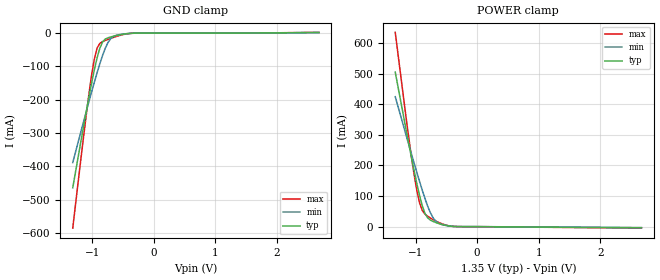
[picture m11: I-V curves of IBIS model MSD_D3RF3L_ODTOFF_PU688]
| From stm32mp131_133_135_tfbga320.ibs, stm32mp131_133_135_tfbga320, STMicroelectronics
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[Model] MSD_D3RF3L_ODTOFF_PU688
Model_type   Input
C_comp 2.455pF   2.369pF   2.579pF
Vinh = 810.000mV
Vinl = 540.000mV
[Receiver Thresholds]
Vth   =  0.675V
Vth_min  =  0.6615V
Vth_max  =  0.6885V
Vinh_ac  =  0.160V
Vinh_dc  =  0.090V
Vinl_ac  = -0.160V
Vinl_dc  = -0.090V
Tslew_ac =  5.000ns |Not specified, so set to high value
[Temperature Range]   25.000   125.000   -40.000
[Voltage Range]   1.350V   1.283V   1.450V
[GND Clamp Reference]   0.00V   0.00V   0.00V
[POWER Clamp Reference]   1.350V   1.283V   1.450V
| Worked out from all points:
|   GND clamp passes 1 mA (typ) near -0.40 V on its own axis
|   POWER clamp passes 1 mA (typ) near -0.41 V on its own axis
[GND Clamp]
-1.318V   -464.2mA   -388.6mA   -585.4mA
-1.142V   -279.7mA   -265.4mA   -310.1mA
-1.055V   -191.2mA   -205.1mA   -181.9mA
-1.011V   -149mA     -175.7mA   -124.8mA
-966.7mV  -109.4mA   -146.8mA   -77.16mA
-922.7mV  -74.06mA   -118.9mA   -44.93mA
-878.8mV  -45.53mA   -92.26mA   -30.7mA
-790.9mV  -17.98mA   -45.94mA   -21.98mA
-703mV    -11.54mA   -16.73mA   -15.85mA
-527.3mV  -4.141mA   -3.476mA   -5.586mA
-307.6mV  -130.2uA   -188uA     -117.4uA
2.68V     1.938mA    1.644mA    2.298mA
[Power Clamp]
-1.33V    504.7mA    424.5mA    634.6mA
-1.111V   271.3mA    268.3mA    290.7mA
-1.023V   181.7mA    206.9mA    168.9mA
-978.8mV  139.7mA    176.9mA    117.6mA
-934.9mV  101mA      147.3mA    77.22mA
-890.9mV  67.93mA    118.7mA    52.77mA
-847mV    43.16mA    91.53mA    40.81mA
-803mV    28.55mA    66.6mA     33.76mA
-715.1mV  16.87mA    28.61mA    22.85mA
-671.2mV  13.34mA    17.63mA    18.15mA
-407.6mV  950.3uA    1.241mA    1.157mA
2.668V    -3.817mA   -3.061mA   -4.926mA
